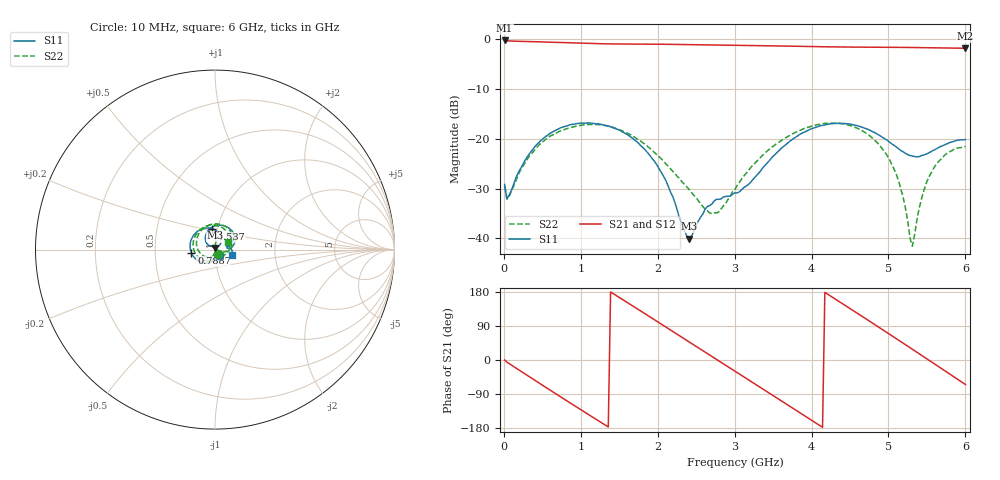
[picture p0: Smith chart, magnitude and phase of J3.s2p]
!Agilent Technologies,E8364B,MY43040528,A.07.50.67
!Agilent E8364B: A.07.50.67
!Date: Sunday, September 28, 2025 22:01:51
!Correction: S11(Full 2 Port(1,2))
!S21(Full 2 Port(1,2))
!S12(Full 2 Port(1,2))
!S22(Full 2 Port(1,2))
!S2P File: Measurements: S11, S21, S12, S22:
# Hz S  dB  R 50
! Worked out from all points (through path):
!   201 points, 10 MHz to 6 GHz, reference 50 ohm
!   highest |S21| = -0.26 dB at 10 MHz (marker M1); lowest = -1.8 dB at 6 GHz (marker M2)
!   group delay of S21, straight-line fit = 361 ps
!   lowest |S11| = -40.1 dB at 2.406 GHz (marker M3), VSWR 1.02, Z = 49.9 + j0.99 ohm
!   |S11| at or under -10 dB: start of sweep to end of sweep
!   |S22| runs from -41.6 to -16.8 dB; largest |S21 - S12| = 0.0074
!   S11 on the Smith chart (normalised r, x): 10 MHz: 1.04, -0.06; 788.7 MHz: 0.77, -0.03; 1.537 GHz: 0.94, +0.22; 6 GHz: 1.20, -0.08
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1e7  -29.18 -52.1  -0.26 -0.1  -0.30 0.2  -29.65 -54.8
3.995e7  -32.05 -37.3  -0.32 -5.6  -0.33 -5.2  -32.16 -39.0
4.293e8  -21.15 -120.7  -0.53 -57.0  -0.52 -56.9  -21.74 -131.2
7.887e8  -17.55 -172.3  -0.71 -103.8  -0.70 -103.7  -18.14 169.8
1.0283e9  -16.85 157.5  -0.83 -134.7  -0.83 -134.6  -17.23 133.1
1.29785e9  -17.25 125.5  -0.93 -169.1  -0.94 -169.0  -17.30 93.0
1.53745e9  -18.60 98.0  -0.98 160.4  -0.98 160.5  -18.37 56.8
2.01665e9  -26.00 49.8  -1.01 98.7  -1.02 98.8  -23.57 -20.9
2.406e9  -40.06 93.7  -1.09 48.2  -1.09 48.3  -30.11 -87.7
2.7055e9  -33.10 130.4  -1.16 9.4  -1.16 9.5  -35.01 -103.7
3.005e9  -30.84 135.5  -1.23 -29.4  -1.22 -29.3  -30.15 -102.5
3.27455e9  -27.56 146.4  -1.29 -64.4  -1.28 -64.3  -24.72 -132.9
3.51415e9  -23.31 139.0  -1.35 -95.6  -1.34 -95.5  -21.36 -167.4
4.0233e9  -17.87 94.7  -1.49 -162.0  -1.49 -161.9  -17.39 118.1
4.29285e9  -16.94 67.3  -1.56 162.9  -1.56 163.1  -16.83 80.9
4.59235e9  -17.38 38.1  -1.60 123.8  -1.60 123.9  -17.89 41.1
5.01165e9  -20.64 7.6  -1.63 68.3  -1.63 68.5  -24.15 -9.9
5.19135e9  -22.63 5.0  -1.65 44.4  -1.65 44.5  -31.82 -23.1
5.31115e9  -23.45 8.7  -1.67 28.3  -1.67 28.5  -41.58 36.2
5.5208e9  -22.87 15.1  -1.72 0.2  -1.72 0.4  -27.83 83.5
5.7604e9  -21.00 5.1  -1.78 -32.1  -1.77 -32.0  -22.95 57.8
6e9  -20.15 -19.4  -1.83 -64.6  -1.83 -64.4  -21.56 31.5
